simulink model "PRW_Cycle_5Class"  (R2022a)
settings: Solver=VariableStepAuto  StartTime=0.0  StopTime=simtime  RelTol=1e-3
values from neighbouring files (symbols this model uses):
  GT = SOH_p01(data_length_finish,1)    [Data_preparation.m]    (also in SimulationCycle.m = 1)
libraries: neural x183
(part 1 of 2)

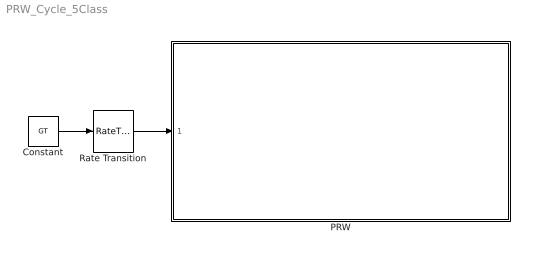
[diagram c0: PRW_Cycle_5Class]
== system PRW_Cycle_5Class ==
  Constant : Constant  Value=GT
  PRW : Subsystem
  Rate Transition : RateTransition  OutPortSampleTime=1
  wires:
  Rate Transition/1 -> PRW/1(SOH)
  Constant/1 -> Rate Transition/1

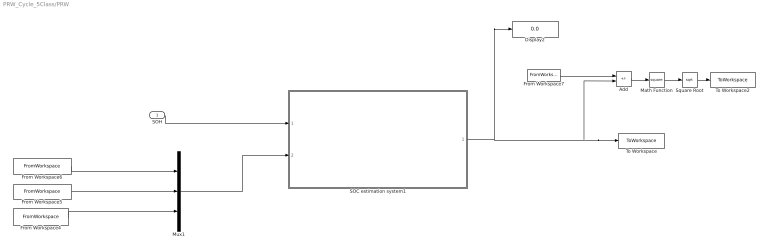
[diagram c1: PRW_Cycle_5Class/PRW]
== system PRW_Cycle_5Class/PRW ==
  SOH : Inport
  Add : Sum  Inputs=+-
  Display2 : Display
  From Workspace4 : FromWorkspace  VariableName=Temperature37
  From Workspace5 : FromWorkspace  VariableName=Voltage37  SampleTime=1
  From Workspace6 : FromWorkspace  VariableName=Current37  SampleTime=1
  From Workspace7 : FromWorkspace  VariableName=SOC_37_GT
  Math Function : Math  Operator=square
  Mux1 : Mux  Inputs=3
  SOC estimation system1 : Subsystem
  Square Root : Sqrt
  To Workspace : ToWorkspace  VariableName=SOC_37_pred  SaveFormat=Timeseries  SampleTime=-1
  To Workspace2 : ToWorkspace  VariableName=SOC_37_abserror  SampleTime=-1
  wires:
  From Workspace6/1 -> Mux1/1
  From Workspace5/1 -> Mux1/2
  From Workspace4/1 -> Mux1/3
  Mux1/1 -> SOC estimation system1/2(Input)
  SOH/1 -> SOC estimation system1/1(Input1)
  Math Function/1 -> Square Root/1
  SOC estimation system1/1(SOC) -> Display2/1, To Workspace/1, Add/2
  From Workspace7/1 -> Add/1
  Add/1 -> Math Function/1
  Square Root/1 -> To Workspace2/1

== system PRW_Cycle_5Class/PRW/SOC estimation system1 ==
  Input1 : Inport
  Input : Inport  Port=2
  Class 1 : Subsystem
  Class 2 : Subsystem
  Class 3 : Subsystem
  Class 4 : Subsystem
  Class 5 : Subsystem
  If1 : If  IfExpression=0.96<u1  ElseIfExpressions=0.92<u1&u1<=0.96  ShowElse=off
  If2 : If  IfExpression=0.9<u1&u1<=0.92  ElseIfExpressions=0.87<u1&u1<=0.9  ShowElse=off
  If3 : If  IfExpression=u1<=0.87  ShowElse=off
  Merge1 : Merge  Inputs=5
  SOC : Outport
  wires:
  If3/1 -> Class 5/Action
  If2/2 -> Class 4/Action
  Class 3/1(Output2) -> Merge1/3
  Class 2/1(Output1) -> Merge1/2
  Class 1/1(Output) -> Merge1/1
  If1/1 -> Class 1/Action
  Class 4/1(Output3) -> Merge1/4
  Input1/1 -> If3/1, If1/1, If2/1
  Class 5/1(Output4) -> Merge1/5
  Merge1/1 -> SOC/1
  If1/2 -> Class 2/Action
  If2/1 -> Class 3/Action
  Input/1 -> Class 1/1(Input), Class 2/1(Input1), Class 3/1(Input2), Class 4/1(Input3), Class 5/1(Input4)

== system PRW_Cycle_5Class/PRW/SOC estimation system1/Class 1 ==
  Input : Inport
  Action Port : ActionPort  ActionPortLabel=if(0.96<u1)
  Class 1-NARX Neural Network : Subsystem  mask{pi_input_1_delayed_1=[0.5037406483790520805854384889244101941585540771484375;0.940456819140602195972178378724493086338043212890625;-0.2518202360030123987399974794243462383747100830078125], ai_layer_2_delayed_1=0.9999911873568390063837796333245933055877685546875}
      mask prompts: pi_input_1_delayed_1 "Preprocessed initial input 1 state at timestep 0."; ai_layer_2_delayed_1 "Initial layer 2 state at timestep 0."
      mask help: NARX Neural Network
  Output : Outport
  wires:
  Class 1-NARX Neural Network/1(y) -> Output/1
  Input/1 -> Class 1-NARX Neural Network/1(x)

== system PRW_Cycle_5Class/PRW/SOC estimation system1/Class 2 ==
  Input1 : Inport
  Action Port : ActionPort  ActionPortLabel=elseif(0.92<u1&u1<=0.96)
  Class2-NARX Neural Network : Subsystem  mask{pi_input_1_delayed_1=[0.4967578681005850871343909602728672325611114501953125;0.9493670886075957771055300327134318649768829345703125;-0.57323420074349396013957402828964404761791229248046875], ai_layer_2_delayed_1=0.99999172247877510244506993331015110015869140625}
      mask prompts: pi_input_1_delayed_1 "Preprocessed initial input 1 state at timestep 0."; ai_layer_2_delayed_1 "Initial layer 2 state at timestep 0."
      mask help: NARX Neural Network
  Output1 : Outport
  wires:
  Input1/1 -> Class2-NARX Neural Network/1(x)
  Class2-NARX Neural Network/1(y) -> Output1/1

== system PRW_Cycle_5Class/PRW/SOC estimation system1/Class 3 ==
  Input2 : Inport
  Action Port : ActionPort  ActionPortLabel=if(0.9<u1&u1<=0.92)
  Class3-NARX Neural Network : Subsystem  mask{pi_input_1_delayed_1=[0.503541633873760385853302068426273763179779052734375;0.9477866061293991339908870941144414246082305908203125;-1.2699044585987255828740671859122812747955322265625], ai_layer_2_delayed_1=0.99999085582048241604979921248741447925567626953125}
      mask prompts: pi_input_1_delayed_1 "Preprocessed initial input 1 state at timestep 0."; ai_layer_2_delayed_1 "Initial layer 2 state at timestep 0."
      mask help: NARX Neural Network
  Output2 : Outport
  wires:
  Class3-NARX Neural Network/1(y) -> Output2/1
  Input2/1 -> Class3-NARX Neural Network/1(x)

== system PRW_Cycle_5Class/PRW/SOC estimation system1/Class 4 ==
  Input3 : Inport
  Action Port : ActionPort  ActionPortLabel=elseif(0.87<u1&u1<=0.9)
  Class 4-NARX Neural Network : Subsystem  mask{pi_input_1_delayed_1=[0.509984639016896945662438156432472169399261474609375;0.9369725738396628145210343063808977603912353515625;-0.6748366013071891433838800367084331810474395751953125], ai_layer_2_delayed_1=0.999984478854660352453720406629145145416259765625}
      mask prompts: pi_input_1_delayed_1 "Preprocessed initial input 1 state at timestep 0."; ai_layer_2_delayed_1 "Initial layer 2 state at timestep 0."
      mask help: NARX Neural Network
  Output3 : Outport
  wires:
  Class 4-NARX Neural Network/1(y) -> Output3/1
  Input3/1 -> Class 4-NARX Neural Network/1(x)

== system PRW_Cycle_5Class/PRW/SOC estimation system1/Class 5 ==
  Input4 : Inport
  Action Port : ActionPort  ActionPortLabel=if(u1<=0.87)
  Class5-NARX Neural Network : Subsystem  mask{pi_input_1_delayed_1=[0.5179502915004601248938342905603349208831787109375;0.9320641543877956625152592096128500998020172119140625;-0.2691648297820226076737526454962790012359619140625], ai_layer_2_delayed_1=0.999983626849760387500509750680066645145416259765625}
      mask prompts: pi_input_1_delayed_1 "Preprocessed initial input 1 state at timestep 0."; ai_layer_2_delayed_1 "Initial layer 2 state at timestep 0."
      mask help: NARX Neural Network
  Output4 : Outport
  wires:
  Class5-NARX Neural Network/1(y) -> Output4/1
  Input4/1 -> Class5-NARX Neural Network/1(x)

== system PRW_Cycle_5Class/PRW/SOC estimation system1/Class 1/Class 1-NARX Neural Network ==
  x : Inport  PortDimensions=3  SampleTime=1
  Layer 1 : Subsystem
  Layer 2 : Subsystem
  Process Input 1 : Subsystem
  Process Output 1 : Subsystem
  y : Outport  InitialOutput=0
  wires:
  x/1 -> Process Input 1/1(x)
  Process Output 1/1(y) -> y/1
  Process Input 1/1(p) -> Layer 1/1("p{1}")
  Layer 1/1("a{1}") -> [feedback1]
  [feedback1] -> Layer 2/1("a{1} ")
  Layer 2/1("a{2}") -> [feedback2], Process Output 1/1(a)
  [feedback2] -> Layer 1/2("a{2} ")

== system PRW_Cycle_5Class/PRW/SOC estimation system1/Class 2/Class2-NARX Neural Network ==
  x : Inport  PortDimensions=3  SampleTime=1
  Layer 1 : Subsystem
  Layer 2 : Subsystem
  Process Input 1 : Subsystem
  Process Output 1 : Subsystem
  y : Outport  InitialOutput=0
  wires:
  x/1 -> Process Input 1/1(x)
  Process Output 1/1(y) -> y/1
  Process Input 1/1(p) -> Layer 1/1("p{1}")
  Layer 1/1("a{1}") -> [feedback1]
  [feedback1] -> Layer 2/1("a{1} ")
  Layer 2/1("a{2}") -> [feedback2], Process Output 1/1(a)
  [feedback2] -> Layer 1/2("a{2} ")

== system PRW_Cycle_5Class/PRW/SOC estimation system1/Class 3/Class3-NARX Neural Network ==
  x : Inport  PortDimensions=3  SampleTime=1
  Layer 1 : Subsystem
  Layer 2 : Subsystem
  Process Input 1 : Subsystem
  Process Output 1 : Subsystem
  y : Outport  InitialOutput=0
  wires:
  x/1 -> Process Input 1/1(x)
  Process Output 1/1(y) -> y/1
  Process Input 1/1(p) -> Layer 1/1("p{1}")
  Layer 1/1("a{1}") -> [feedback1]
  [feedback1] -> Layer 2/1("a{1} ")
  Layer 2/1("a{2}") -> [feedback2], Process Output 1/1(a)
  [feedback2] -> Layer 1/2("a{2} ")

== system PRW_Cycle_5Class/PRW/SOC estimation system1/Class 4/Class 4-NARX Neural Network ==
  x : Inport  PortDimensions=3  SampleTime=1
  Layer 1 : Subsystem
  Layer 2 : Subsystem
  Process Input 1 : Subsystem
  Process Output 1 : Subsystem
  y : Outport  InitialOutput=0
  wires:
  x/1 -> Process Input 1/1(x)
  Process Output 1/1(y) -> y/1
  Process Input 1/1(p) -> Layer 1/1("p{1}")
  Layer 1/1("a{1}") -> [feedback1]
  [feedback1] -> Layer 2/1("a{1} ")
  Layer 2/1("a{2}") -> [feedback2], Process Output 1/1(a)
  [feedback2] -> Layer 1/2("a{2} ")

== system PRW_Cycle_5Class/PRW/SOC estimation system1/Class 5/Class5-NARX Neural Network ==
  x : Inport  PortDimensions=3  SampleTime=1
  Layer 1 : Subsystem
  Layer 2 : Subsystem
  Process Input 1 : Subsystem
  Process Output 1 : Subsystem
  y : Outport  InitialOutput=0
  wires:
  x/1 -> Process Input 1/1(x)
  Process Output 1/1(y) -> y/1
  Process Input 1/1(p) -> Layer 1/1("p{1}")
  Layer 1/1("a{1}") -> [feedback1]
  [feedback1] -> Layer 2/1("a{1} ")
  Layer 2/1("a{2}") -> [feedback2], Process Output 1/1(a)
  [feedback2] -> Layer 1/2("a{2} ")

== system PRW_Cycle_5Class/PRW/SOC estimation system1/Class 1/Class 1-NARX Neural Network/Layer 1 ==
  "p{1}" : Inport  PortDimensions=3  SampleTime=1
  "a{2} " : Inport  Port=2  PortDimensions=1  SampleTime=1
  Delays 1 : Subsystem
  Delays 2 : Subsystem
  "IW{1,1}" : Subsystem
  "LW{1,2}" : Subsystem
  "b{1}" : Constant  Value=[2.34272603015963820638489778502844274044036865234375;-1.83098571478465554918102498049847781658172607421875;-0.79131154125893576889438918442465364933013916015625;-1.2076273263687624659468156096409074962139129638671875;0.84071386902655909079129514793748967349529266357421875;-0.53056878404548457606182410017936490476131439208984375;-0.0240383625943490740473063027593525475822389125823974609375;0.16604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
  netsum : Sum  Inputs=3  InputSameDT=on  SaturateOnIntegerOverflow=on
  tansig : neural/Transfer Functions/tansig
  "a{1}" : Outport  InitialOutput=[0;0;0;0;0;0;0;0;0;0;0;0;0;0;0]
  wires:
  "p{1}"/1 -> Delays 1/1("p{1}")
  Delays 1/1("pd{1,1}") -> "IW{1,1}"/1("pd{1,1}")
  "IW{1,1}"/1("iz{1,1}") -> netsum/1
  "a{2} "/1 -> Delays 2/1("p{1}")
  Delays 2/1("pd{1,2}") -> "LW{1,2}"/1("ad{1,2}")
  "LW{1,2}"/1("lz{1,2}") -> netsum/2
  "b{1}"/1 -> netsum/3
  netsum/1 -> tansig/1
  tansig/1 -> "a{1}"/1

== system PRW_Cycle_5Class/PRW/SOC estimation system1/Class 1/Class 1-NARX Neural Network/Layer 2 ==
  "a{1} " : Inport  PortDimensions=15  SampleTime=1
  Delays 1 : Subsystem
  "LW{2,1}" : Subsystem
  "b{2}" : Constant  Value=-0.2610570456976468722842810166184790432453155517578125
  netsum : Sum  Inputs=2  InputSameDT=on  SaturateOnIntegerOverflow=on
  purelin : neural/Transfer Functions/purelin
  "a{2}" : Outport  InitialOutput=0
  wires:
  "a{1} "/1 -> Delays 1/1("p{2}")
  Delays 1/1("pd{2,1}") -> "LW{2,1}"/1("ad{2,1}")
  "LW{2,1}"/1("lz{2,1}") -> netsum/1
  "b{2}"/1 -> netsum/2
  netsum/1 -> purelin/1
  purelin/1 -> "a{2}"/1

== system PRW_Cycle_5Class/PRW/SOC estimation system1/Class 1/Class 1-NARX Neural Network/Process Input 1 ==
  x : Inport  PortDimensions=3  SampleTime=1
  mapminmax : neural/Processing Functions/mapminmax  xmin=[-4.82500000000000017763568394003;2.50570000000000003836930773105;17.1380000000000016768808563938]  xmax=[1.5909999999999999698019337302;4.16500000000000003552713678801;25.1039999999999992041921359487]  ymin=-1  ymax=1
  p : Outport  PortDimensions=3  SampleTime=1
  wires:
  x/1 -> mapminmax/1
  mapminmax/1 -> p/1

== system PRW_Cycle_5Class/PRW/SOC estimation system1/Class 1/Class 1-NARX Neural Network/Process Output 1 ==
  a : Inport  PortDimensions=1  SampleTime=1
  mapminmax_reverse : neural/Processing Functions/mapminmax_reverse  xmin=-2.62341179120179950748424461959e-06  xmax=1.00000440635255594123975697585  ymin=-1  ymax=1
  y : Outport  PortDimensions=1  SampleTime=1
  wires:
  a/1 -> mapminmax_reverse/1
  mapminmax_reverse/1 -> y/1

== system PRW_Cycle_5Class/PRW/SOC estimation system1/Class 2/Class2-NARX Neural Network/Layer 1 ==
  "p{1}" : Inport  PortDimensions=3  SampleTime=1
  "a{2} " : Inport  Port=2  PortDimensions=1  SampleTime=1
  Delays 1 : Subsystem
  Delays 2 : Subsystem
  "IW{1,1}" : Subsystem
  "LW{1,2}" : Subsystem
  "b{1}" : Constant  Value=[2.123679128509173619221428452874533832073211669921875;-2.87621199885181422217783619998954236507415771484375;-0.54420836494168567387674784185946919023990631103515625;-0.5394065908795988573132262899889610707759857177734375;0.85139936745729760669831875929958187043666839599609375;-1.1563643607811477931335275570745579898357391357421875;-0.61089692546734919442741329476120881736278533935546875;-0.197690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
  netsum : Sum  Inputs=3  InputSameDT=on  SaturateOnIntegerOverflow=on
  tansig : neural/Transfer Functions/tansig
  "a{1}" : Outport  InitialOutput=[0;0;0;0;0;0;0;0;0;0;0;0;0;0;0;0]
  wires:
  "p{1}"/1 -> Delays 1/1("p{1}")
  Delays 1/1("pd{1,1}") -> "IW{1,1}"/1("pd{1,1}")
  "IW{1,1}"/1("iz{1,1}") -> netsum/1
  "a{2} "/1 -> Delays 2/1("p{1}")
  Delays 2/1("pd{1,2}") -> "LW{1,2}"/1("ad{1,2}")
  "LW{1,2}"/1("lz{1,2}") -> netsum/2
  "b{1}"/1 -> netsum/3
  netsum/1 -> tansig/1
  tansig/1 -> "a{1}"/1

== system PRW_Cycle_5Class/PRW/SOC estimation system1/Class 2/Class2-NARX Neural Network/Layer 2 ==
  "a{1} " : Inport  PortDimensions=16  SampleTime=1
  Delays 1 : Subsystem
  "LW{2,1}" : Subsystem
  "b{2}" : Constant  Value=0.1380564376019000061290853409445844590663909912109375
  netsum : Sum  Inputs=2  InputSameDT=on  SaturateOnIntegerOverflow=on
  purelin : neural/Transfer Functions/purelin
  "a{2}" : Outport  InitialOutput=0
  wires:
  "a{1} "/1 -> Delays 1/1("p{2}")
  Delays 1/1("pd{2,1}") -> "LW{2,1}"/1("ad{2,1}")
  "LW{2,1}"/1("lz{2,1}") -> netsum/1
  "b{2}"/1 -> netsum/2
  netsum/1 -> purelin/1
  purelin/1 -> "a{2}"/1

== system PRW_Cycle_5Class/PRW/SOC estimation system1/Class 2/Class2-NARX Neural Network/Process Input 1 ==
  x : Inport  PortDimensions=3  SampleTime=1
  mapminmax : neural/Processing Functions/mapminmax  xmin=[-4.73300000000000054001247917768;2.63719999999999998863131622784;17.8219999999999991757704265183]  xmax=[1.59000000000000007993605777301;4.15399999999999991473487170879;28.5820000000000007389644451905]  ymin=-1  ymax=1
  p : Outport  PortDimensions=3  SampleTime=1
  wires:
  x/1 -> mapminmax/1
  mapminmax/1 -> p/1

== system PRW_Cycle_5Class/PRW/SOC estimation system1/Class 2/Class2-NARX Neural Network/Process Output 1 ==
  a : Inport  PortDimensions=1  SampleTime=1
  mapminmax_reverse : neural/Processing Functions/mapminmax_reverse  xmin=-3.32617917940104848405083806662e-06  xmax=1.00000413879150817919594373961  ymin=-1  ymax=1
  y : Outport  PortDimensions=1  SampleTime=1
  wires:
  a/1 -> mapminmax_reverse/1
  mapminmax_reverse/1 -> y/1

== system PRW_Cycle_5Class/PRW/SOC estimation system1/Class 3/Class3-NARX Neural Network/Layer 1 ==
  "p{1}" : Inport  PortDimensions=3  SampleTime=1
  "a{2} " : Inport  Port=2  PortDimensions=1  SampleTime=1
  Delays 1 : Subsystem
  Delays 2 : Subsystem
  "IW{1,1}" : Subsystem
  "LW{1,2}" : Subsystem
  "b{1}" : Constant  Value=[-1.93346371221756019309623297885991632938385009765625;1.7923652112547914239115698364912532269954681396484375;1.1238522489621971534035083095659501850605010986328125;0.323356733008480279334406759517150931060314178466796875;0.76493308526969572280762577065615914762020111083984375;-0.351089604850296443938617585445172153413295745849609375;0.33583797370279000471526842375169508159160614013671875;-0.46332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
  netsum : Sum  Inputs=3  InputSameDT=on  SaturateOnIntegerOverflow=on
  tansig : neural/Transfer Functions/tansig
  "a{1}" : Outport  InitialOutput=[0;0;0;0;0;0;0;0;0;0;0;0;0;0;0]
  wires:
  "p{1}"/1 -> Delays 1/1("p{1}")
  Delays 1/1("pd{1,1}") -> "IW{1,1}"/1("pd{1,1}")
  "IW{1,1}"/1("iz{1,1}") -> netsum/1
  "a{2} "/1 -> Delays 2/1("p{1}")
  Delays 2/1("pd{1,2}") -> "LW{1,2}"/1("ad{1,2}")
  "LW{1,2}"/1("lz{1,2}") -> netsum/2
  "b{1}"/1 -> netsum/3
  netsum/1 -> tansig/1
  tansig/1 -> "a{1}"/1

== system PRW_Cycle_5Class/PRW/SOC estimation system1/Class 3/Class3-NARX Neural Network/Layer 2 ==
  "a{1} " : Inport  PortDimensions=15  SampleTime=1
  Delays 1 : Subsystem
  "LW{2,1}" : Subsystem
  "b{2}" : Constant  Value=0.272834520121191526076387390276067890226840972900390625
  netsum : Sum  Inputs=2  InputSameDT=on  SaturateOnIntegerOverflow=on
  purelin : neural/Transfer Functions/purelin
  "a{2}" : Outport  InitialOutput=0
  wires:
  "a{1} "/1 -> Delays 1/1("p{2}")
  Delays 1/1("pd{2,1}") -> "LW{2,1}"/1("ad{2,1}")
  "LW{2,1}"/1("lz{2,1}") -> netsum/1
  "b{2}"/1 -> netsum/2
  netsum/1 -> purelin/1
  purelin/1 -> "a{2}"/1

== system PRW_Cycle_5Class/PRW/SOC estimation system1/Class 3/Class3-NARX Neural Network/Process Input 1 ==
  x : Inport  PortDimensions=3  SampleTime=1
  mapminmax : neural/Processing Functions/mapminmax  xmin=[-4.77700000000000013500311979442;2.6570000000000000284217094304;21.4740000000000001989519660128]  xmax=[1.57600000000000006750155989721;4.15470000000000005968558980385;31.5220000000000020179413695587]  ymin=-1  ymax=1
  p : Outport  PortDimensions=3  SampleTime=1
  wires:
  x/1 -> mapminmax/1
  mapminmax/1 -> p/1

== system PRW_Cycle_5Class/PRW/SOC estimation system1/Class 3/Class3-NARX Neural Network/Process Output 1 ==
  a : Inport  PortDimensions=1  SampleTime=1
  mapminmax_reverse : neural/Processing Functions/mapminmax_reverse  xmin=-3.07535918984610110574521267546e-06  xmax=1.00000457212472371182343522378  ymin=-1  ymax=1
  y : Outport  PortDimensions=1  SampleTime=1
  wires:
  a/1 -> mapminmax_reverse/1
  mapminmax_reverse/1 -> y/1

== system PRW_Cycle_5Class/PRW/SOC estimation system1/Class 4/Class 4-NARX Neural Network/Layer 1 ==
  "p{1}" : Inport  PortDimensions=3  SampleTime=1
  "a{2} " : Inport  Port=2  PortDimensions=1  SampleTime=1
  Delays 1 : Subsystem
  Delays 2 : Subsystem
  "IW{1,1}" : Subsystem
  "LW{1,2}" : Subsystem
  "b{1}" : Constant  Value=[-2.688444044962437828871770761907100677490234375;0.858381113224772729353162503684870898723602294921875;-2.222715747204785596835563410422764718532562255859375;1.3209762857863693863436083120177499949932098388671875;-0.8915787953875426996575015436974354088306427001953125;-0.88615966223780884281069347707671113312244415283203125;0.280218393721010927688297442728071473538875579833984375;0.21524348971530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
  netsum : Sum  Inputs=3  InputSameDT=on  SaturateOnIntegerOverflow=on
  tansig : neural/Transfer Functions/tansig
  "a{1}" : Outport  InitialOutput=[0;0;0;0;0;0;0;0;0;0;0;0;0;0;0]
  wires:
  "p{1}"/1 -> Delays 1/1("p{1}")
  Delays 1/1("pd{1,1}") -> "IW{1,1}"/1("pd{1,1}")
  "IW{1,1}"/1("iz{1,1}") -> netsum/1
  "a{2} "/1 -> Delays 2/1("p{1}")
  Delays 2/1("pd{1,2}") -> "LW{1,2}"/1("ad{1,2}")
  "LW{1,2}"/1("lz{1,2}") -> netsum/2
  "b{1}"/1 -> netsum/3
  netsum/1 -> tansig/1
  tansig/1 -> "a{1}"/1

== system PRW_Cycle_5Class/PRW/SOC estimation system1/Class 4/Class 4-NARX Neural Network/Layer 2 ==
  "a{1} " : Inport  PortDimensions=15  SampleTime=1
  Delays 1 : Subsystem
  "LW{2,1}" : Subsystem
  "b{2}" : Constant  Value=0.045626078950611735629561138694043620489537715911865234375
  netsum : Sum  Inputs=2  InputSameDT=on  SaturateOnIntegerOverflow=on
  purelin : neural/Transfer Functions/purelin
  "a{2}" : Outport  InitialOutput=0
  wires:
  "a{1} "/1 -> Delays 1/1("p{2}")
  Delays 1/1("pd{2,1}") -> "LW{2,1}"/1("ad{2,1}")
  "LW{2,1}"/1("lz{2,1}") -> netsum/1
  "b{2}"/1 -> netsum/2
  netsum/1 -> purelin/1
  purelin/1 -> "a{2}"/1

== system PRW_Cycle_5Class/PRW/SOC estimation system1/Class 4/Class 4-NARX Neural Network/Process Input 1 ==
  x : Inport  PortDimensions=3  SampleTime=1
  mapminmax : neural/Processing Functions/mapminmax  xmin=[-4.91600000000000036948222259525;2.64660000000000028563817977556;18.5259999999999998010480339872]  xmax=[1.59400000000000008348877145181;4.16340000000000021174173525651;28.3180000000000013926637620898]  ymin=-1  ymax=1
  p : Outport  PortDimensions=3  SampleTime=1
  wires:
  x/1 -> mapminmax/1
  mapminmax/1 -> p/1

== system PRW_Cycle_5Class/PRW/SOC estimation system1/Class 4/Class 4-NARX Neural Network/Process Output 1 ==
  a : Inport  PortDimensions=1  SampleTime=1
  mapminmax_reverse : neural/Processing Functions/mapminmax_reverse  xmin=-4.21949321457851519659313158095e-06  xmax=1.00000776066564278643511443079  ymin=-1  ymax=1
  y : Outport  PortDimensions=1  SampleTime=1
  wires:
  a/1 -> mapminmax_reverse/1
  mapminmax_reverse/1 -> y/1

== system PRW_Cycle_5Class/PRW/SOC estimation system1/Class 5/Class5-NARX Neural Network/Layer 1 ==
  "p{1}" : Inport  PortDimensions=3  SampleTime=1
  "a{2} " : Inport  Port=2  PortDimensions=1  SampleTime=1
  Delays 1 : Subsystem
  Delays 2 : Subsystem
  "IW{1,1}" : Subsystem
  "LW{1,2}" : Subsystem
  "b{1}" : Constant  Value=[-1.9239326886795684590225619103875942528247833251953125;-1.4156259333430829538968964698142372071743011474609375;-1.8809744346361843003734293233719654381275177001953125;-1.106968201899322767900457620271481573581695556640625;1.16695809702027997190043606678955256938934326171875;1.0579085603689832861817876619170419871807098388671875;0.33221840417104486764543480603606440126895904541015625;-0.035398306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
  netsum : Sum  Inputs=3  InputSameDT=on  SaturateOnIntegerOverflow=on
  tansig : neural/Transfer Functions/tansig
  "a{1}" : Outport  InitialOutput=[0;0;0;0;0;0;0;0;0;0;0;0;0;0;0;0;0;0]
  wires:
  "p{1}"/1 -> Delays 1/1("p{1}")
  Delays 1/1("pd{1,1}") -> "IW{1,1}"/1("pd{1,1}")
  "IW{1,1}"/1("iz{1,1}") -> netsum/1
  "a{2} "/1 -> Delays 2/1("p{1}")
  Delays 2/1("pd{1,2}") -> "LW{1,2}"/1("ad{1,2}")
  "LW{1,2}"/1("lz{1,2}") -> netsum/2
  "b{1}"/1 -> netsum/3
  netsum/1 -> tansig/1
  tansig/1 -> "a{1}"/1

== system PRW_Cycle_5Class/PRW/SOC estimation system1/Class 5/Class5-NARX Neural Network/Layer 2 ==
  "a{1} " : Inport  PortDimensions=18  SampleTime=1
  Delays 1 : Subsystem
  "LW{2,1}" : Subsystem
  "b{2}" : Constant  Value=0.2439901834476533026840883167096762917935848236083984375
  netsum : Sum  Inputs=2  InputSameDT=on  SaturateOnIntegerOverflow=on
  purelin : neural/Transfer Functions/purelin
  "a{2}" : Outport  InitialOutput=0
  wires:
  "a{1} "/1 -> Delays 1/1("p{2}")
  Delays 1/1("pd{2,1}") -> "LW{2,1}"/1("ad{2,1}")
  "LW{2,1}"/1("lz{2,1}") -> netsum/1
  "b{2}"/1 -> netsum/2
  netsum/1 -> purelin/1
  purelin/1 -> "a{2}"/1

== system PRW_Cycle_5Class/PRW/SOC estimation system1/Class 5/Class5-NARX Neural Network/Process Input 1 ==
  x : Inport  PortDimensions=3  SampleTime=1
  mapminmax : neural/Processing Functions/mapminmax  xmin=[-4.94800000000000039790393202566;2.6339000000000001300293206441;17.1340000000000003410605131648]  xmax=[1.57000000000000006217248937901;4.16769999999999996020960679743;25.3000000000000007105427357601]  ymin=-1  ymax=1
  p : Outport  PortDimensions=3  SampleTime=1
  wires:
  x/1 -> mapminmax/1
  mapminmax/1 -> p/1

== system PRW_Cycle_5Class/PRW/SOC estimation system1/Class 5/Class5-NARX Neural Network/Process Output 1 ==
  a : Inport  PortDimensions=1  SampleTime=1
  mapminmax_reverse : neural/Processing Functions/mapminmax_reverse  xmin=-3.87764264893447179729721319141e-06  xmax=1.0000081866738852465203990505  ymin=-1  ymax=1
  y : Outport  PortDimensions=1  SampleTime=1
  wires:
  a/1 -> mapminmax_reverse/1
  mapminmax_reverse/1 -> y/1

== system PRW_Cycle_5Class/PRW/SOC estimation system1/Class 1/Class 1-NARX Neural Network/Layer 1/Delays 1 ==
  "p{1}" : Inport  PortDimensions=3  SampleTime=1
  Delay 1 : UnitDelay  InitialCondition=pi_input_1_delayed_1
  mux : Mux  Inputs=2
  "pd{1,1}" : Outport
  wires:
  "p{1}"/1 -> Delay 1/1, mux/1
  Delay 1/1 -> mux/2
  mux/1 -> "pd{1,1}"/1

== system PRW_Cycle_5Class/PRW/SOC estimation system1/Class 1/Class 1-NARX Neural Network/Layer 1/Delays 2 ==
  "p{1}" : Inport  PortDimensions=1  SampleTime=1
  Delay 1 : UnitDelay  InitialCondition=ai_layer_2_delayed_1
  mux : Mux  Inputs=1
  "pd{1,2}" : Outport
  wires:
  "p{1}"/1 -> Delay 1/1
  Delay 1/1 -> mux/1
  mux/1 -> "pd{1,2}"/1

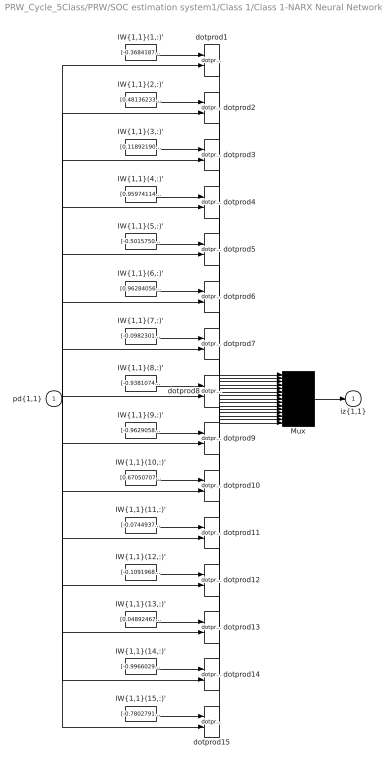
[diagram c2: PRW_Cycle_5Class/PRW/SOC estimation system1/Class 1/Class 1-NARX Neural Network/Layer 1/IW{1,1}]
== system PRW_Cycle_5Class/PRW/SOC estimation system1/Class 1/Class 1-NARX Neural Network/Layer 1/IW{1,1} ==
  "pd{1,1}" : Inport  PortDimensions=6  SampleTime=1
  "IW{1,1}(1,:)'" : Constant  Value=[-0.36841871672555603911547450479702092707157135009765625;0.95481863811988365586813642948982305824756622314453125;0.226878529936702599822950787711306475102901458740234375;0.036258766201381888161225930389264249242842197418212890625;0.3238678699587700382522825748310424387454986572265625;-0.84200791510325945221637766735511831939220428466796875]
  "IW{1,1}(10,:)'" : Constant  Value=[0.67050707720070523709665621936437673866748809814453125;0.882956797146274841026070134830661118030548095703125;-0.90123173513004661838721176536637358367443084716796875;0.89515060785826994216307639362639747560024261474609375;-0.805115591223422466526926655205897986888885498046875;-0.2593277792147092863928037331788800656795501708984375]
  "IW{1,1}(11,:)'" : Constant  Value=[-0.0744937388110009646169373809243552386760711669921875;0.91481150331324145863476360318600200116634368896484375;-0.0033589550935993598736184484465638888650573790073394775390625;0.09387686590177278522784121150834835134446620941162109375;-0.99451251190708223059999681936460547149181365966796875;-0.0003307952570151217433665202793946491510723717510700225830078125]
  "IW{1,1}(12,:)'" : Constant  Value=[-0.10919681936643919895058019164935103617608547210693359375;0.50465640273350442779332070131204091012477874755859375;0.00167935474555881941553792113808185604284517467021942138671875;0.090898075716160431358758842179668135941028594970703125;-0.421892519785072861449037873171619139611721038818359375;0.004083310809217589355812894069686080911196768283843994140625]
  "IW{1,1}(13,:)'" : Constant  Value=[0.048924672243263016280234722898967447690665721893310546875;-0.53987449057316327927225074745365418493747711181640625;0.00170226104659932341023331758833592175506055355072021484375;-0.058328940083118230308656393390265293419361114501953125;0.57776802472895305573530322362785227596759796142578125;-0.00015032127929270978146554516019506309021380729973316192626953125]
  "IW{1,1}(14,:)'" : Constant  Value=[-0.99660291683138291229937522075488232076168060302734375;0.5911312952433938061602702873642556369304656982421875;1.14540739846979366944879075163044035434722900390625;-0.3381076514679877131897001163451932370662689208984375;0.45894832786268346946911833583726547658443450927734375;-0.70176558995015925201954587464570067822933197021484375]
  "IW{1,1}(15,:)'" : Constant  Value=[-0.7802791008156886309876654195250011980533599853515625;1.0534129951958177695559015774051658809185028076171875;-0.03448938205268679835224787666447809897363185882568359375;0.94691798651251091190061970337410457432270050048828125;0.0231481724065754346231216231899452395737171173095703125;-0.5027468755563602176295034951181150972843170166015625]
  "IW{1,1}(2,:)'" : Constant  Value=[0.481362338278815193870485700244898907840251922607421875;-1.50652710762162467261759957182221114635467529296875;-0.2359262305730511488643941220288979820907115936279296875;-0.1406423235510661229330509058854659087955951690673828125;0.1819515858690983478584968224822659976780414581298828125;0.86381133633920403891437445054179988801479339599609375]
  "IW{1,1}(3,:)'" : Constant  Value=[0.11892190500532838492997456114608212374150753021240234375;-0.24493184734591633144873412675224244594573974609375;-0.00451567345059881997126893793392810039222240447998046875;-0.08059998953516155084653149742734967730939388275146484375;0.07911717353434512267629230564125464297831058502197265625;-0.00710306128001607188504618051183570059947669506072998046875]
  "IW{1,1}(4,:)'" : Constant  Value=[0.95974114664550247422170059508061967790126800537109375;-0.8796676994389194259582609447534196078777313232421875;0.9728248784750912481200657566660083830356597900390625;-0.70361057504988477884211306445649825036525726318359375;0.6194834636783788095470981716061942279338836669921875;0.61913161067906596901622151563060469925403594970703125]
  "IW{1,1}(5,:)'" : Constant  Value=[-0.50157500574550883953861557529307901859283447265625;-0.375530160518852185180804781339247711002826690673828125;0.01501545548960662480875161151061547570861876010894775390625;0.757425535532789684367571680922992527484893798828125;-0.77182219089220105434634433549945242702960968017578125;-0.0759994756633779744436907321869512088596820831298828125]
  "IW{1,1}(6,:)'" : Constant  Value=[0.9628405697273880736730689022806473076343536376953125;-0.632510343955252185565996114746667444705963134765625;0.35396101720878470064945986450766213238239288330078125;-0.60680374926630076259925772319547832012176513671875;0.177448918867727456483152082000742666423320770263671875;0.9817426047833206492754243299714289605617523193359375]
  "IW{1,1}(7,:)'" : Constant  Value=[-0.09823010496840246796868001410985016264021396636962890625;-1.185310142409820688413901734747923910617828369140625;0.1908758613743539445106733865031856112182140350341796875;-1.1914761953630537139048328754142858088016510009765625;0.39827398536536140483121926081366837024688720703125;0.90973345961705021078813615531544201076030731201171875]
  "IW{1,1}(8,:)'" : Constant  Value=[-0.93810741037665390518185404289397411048412322998046875;-1.2595077433783707920866845597629435360431671142578125;-0.78652190025548751606265795999206602573394775390625;-0.7895482370616810907648641659761779010295867919921875;0.24445192827118944478570483624935150146484375;0.34046059489771918205036627114168368279933929443359375]
  "IW{1,1}(9,:)'" : Constant  Value=[-0.962905875728648386058239339035935699939727783203125;-0.99822741054854535747153931879438459873199462890625;1.4514584750111370059499904527910985052585601806640625;-0.338753693920172793685452461431850679218769073486328125;-0.2495656714555981314784816049723303876817226409912109375;-0.0823827548058631842220478347371681593358516693115234375]
  Mux : Mux  Inputs=15
  dotprod{1..15} (15 alike) : neural/Weight Functions/dotprod
  "iz{1,1}" : Outport
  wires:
  "IW{1,1}(1,:)'"/1 -> dotprod1/1
  "pd{1,1}"/1 -> dotprod1/2, dotprod2/2, dotprod3/2, dotprod4/2, dotprod5/2, dotprod6/2, dotprod7/2, dotprod8/2, dotprod9/2, dotprod10/2, dotprod11/2, dotprod12/2, dotprod13/2, dotprod14/2, dotprod15/2
  dotprod1/1 -> Mux/1
  "IW{1,1}(2,:)'"/1 -> dotprod2/1
  dotprod2/1 -> Mux/2
  "IW{1,1}(3,:)'"/1 -> dotprod3/1
  dotprod3/1 -> Mux/3
  "IW{1,1}(4,:)'"/1 -> dotprod4/1
  dotprod4/1 -> Mux/4
  "IW{1,1}(5,:)'"/1 -> dotprod5/1
  dotprod5/1 -> Mux/5
  "IW{1,1}(6,:)'"/1 -> dotprod6/1
  dotprod6/1 -> Mux/6
  "IW{1,1}(7,:)'"/1 -> dotprod7/1
  dotprod7/1 -> Mux/7
  "IW{1,1}(8,:)'"/1 -> dotprod8/1
  dotprod8/1 -> Mux/8
  "IW{1,1}(9,:)'"/1 -> dotprod9/1
  dotprod9/1 -> Mux/9
  "IW{1,1}(10,:)'"/1 -> dotprod10/1
  dotprod10/1 -> Mux/10
  "IW{1,1}(11,:)'"/1 -> dotprod11/1
  dotprod11/1 -> Mux/11
  "IW{1,1}(12,:)'"/1 -> dotprod12/1
  dotprod12/1 -> Mux/12
  "IW{1,1}(13,:)'"/1 -> dotprod13/1
  dotprod13/1 -> Mux/13
  "IW{1,1}(14,:)'"/1 -> dotprod14/1
  dotprod14/1 -> Mux/14
  "IW{1,1}(15,:)'"/1 -> dotprod15/1
  dotprod15/1 -> Mux/15
  Mux/1 -> "iz{1,1}"/1

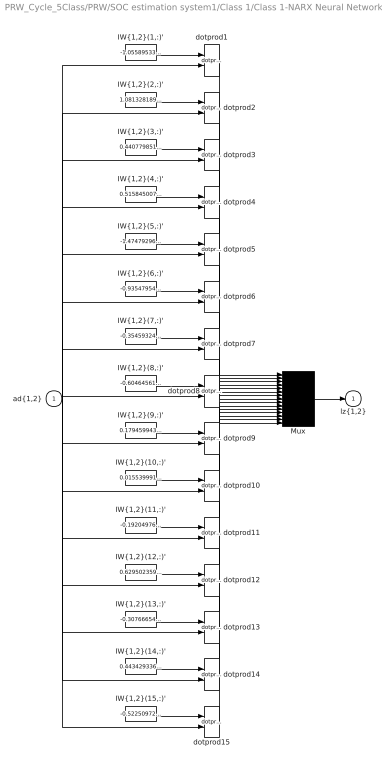
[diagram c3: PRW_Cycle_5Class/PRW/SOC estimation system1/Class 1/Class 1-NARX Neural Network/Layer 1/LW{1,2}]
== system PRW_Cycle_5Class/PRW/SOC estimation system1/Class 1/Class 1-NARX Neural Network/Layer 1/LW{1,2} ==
  "ad{1,2}" : Inport  PortDimensions=1  SampleTime=1
  "IW{1,2}(1,:)'" : Constant  Value=-1.0558953399790829141835502014146186411380767822265625
  "IW{1,2}(10,:)'" : Constant  Value=0.0155399911340668960002542320353313698433339595794677734375
  "IW{1,2}(11,:)'" : Constant  Value=-0.1920497660372149917318296274970634840428829193115234375
  "IW{1,2}(12,:)'" : Constant  Value=0.62950235962305978176800635992549359798431396484375
  "IW{1,2}(13,:)'" : Constant  Value=-0.30766654353943623245726257664500735700130462646484375
  "IW{1,2}(14,:)'" : Constant  Value=0.443429336021788522703701573846046812832355499267578125
  "IW{1,2}(15,:)'" : Constant  Value=-0.52250972552172625373856362784863449633121490478515625
  "IW{1,2}(2,:)'" : Constant  Value=1.08132818981622680354348631226457655429840087890625
  "IW{1,2}(3,:)'" : Constant  Value=0.440779851117324483755766095782746560871601104736328125
  "IW{1,2}(4,:)'" : Constant  Value=0.51584500712902159325068396356073208153247833251953125
  "IW{1,2}(5,:)'" : Constant  Value=-1.47479296662152048469351939274929463863372802734375
  "IW{1,2}(6,:)'" : Constant  Value=-0.935479542831488597443012622534297406673431396484375
  "IW{1,2}(7,:)'" : Constant  Value=-0.354593245240020948916281895435531623661518096923828125
  "IW{1,2}(8,:)'" : Constant  Value=-0.6046456148812133779557598245446570217609405517578125
  "IW{1,2}(9,:)'" : Constant  Value=0.1794599438126181223385202656572801060974597930908203125
  Mux : Mux  Inputs=15
  dotprod{1..15} (15 alike) : neural/Weight Functions/dotprod
  "lz{1,2}" : Outport
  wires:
  "IW{1,2}(1,:)'"/1 -> dotprod1/1
  "ad{1,2}"/1 -> dotprod1/2, dotprod2/2, dotprod3/2, dotprod4/2, dotprod5/2, dotprod6/2, dotprod7/2, dotprod8/2, dotprod9/2, dotprod10/2, dotprod11/2, dotprod12/2, dotprod13/2, dotprod14/2, dotprod15/2
  dotprod1/1 -> Mux/1
  "IW{1,2}(2,:)'"/1 -> dotprod2/1
  dotprod2/1 -> Mux/2
  "IW{1,2}(3,:)'"/1 -> dotprod3/1
  dotprod3/1 -> Mux/3
  "IW{1,2}(4,:)'"/1 -> dotprod4/1
  dotprod4/1 -> Mux/4
  "IW{1,2}(5,:)'"/1 -> dotprod5/1
  dotprod5/1 -> Mux/5
  "IW{1,2}(6,:)'"/1 -> dotprod6/1
  dotprod6/1 -> Mux/6
  "IW{1,2}(7,:)'"/1 -> dotprod7/1
  dotprod7/1 -> Mux/7
  "IW{1,2}(8,:)'"/1 -> dotprod8/1
  dotprod8/1 -> Mux/8
  "IW{1,2}(9,:)'"/1 -> dotprod9/1
  dotprod9/1 -> Mux/9
  "IW{1,2}(10,:)'"/1 -> dotprod10/1
  dotprod10/1 -> Mux/10
  "IW{1,2}(11,:)'"/1 -> dotprod11/1
  dotprod11/1 -> Mux/11
  "IW{1,2}(12,:)'"/1 -> dotprod12/1
  dotprod12/1 -> Mux/12
  "IW{1,2}(13,:)'"/1 -> dotprod13/1
  dotprod13/1 -> Mux/13
  "IW{1,2}(14,:)'"/1 -> dotprod14/1
  dotprod14/1 -> Mux/14
  "IW{1,2}(15,:)'"/1 -> dotprod15/1
  dotprod15/1 -> Mux/15
  Mux/1 -> "lz{1,2}"/1

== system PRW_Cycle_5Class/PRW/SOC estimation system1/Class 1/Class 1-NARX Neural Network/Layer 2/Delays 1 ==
  "p{2}" : Inport  PortDimensions=15  SampleTime=1
  mux : Mux  Inputs=1
  "pd{2,1}" : Outport
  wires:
  "p{2}"/1 -> mux/1
  mux/1 -> "pd{2,1}"/1

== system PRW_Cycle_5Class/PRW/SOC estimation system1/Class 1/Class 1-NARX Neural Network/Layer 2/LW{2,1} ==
  "ad{2,1}" : Inport  PortDimensions=15  SampleTime=1
  "IW{2,1}(1,:)'" : Constant  Value=[-0.4054339128384827350970454062917269766330718994140625;-0.150291660026959761342624233293463476002216339111328125;0.399718217310838286326912793811061419546604156494140625;3.55968054837466467703495365260124572159838862717151641845703125e-05;-0.0023970249922561893095307450352038358687423169612884521484375;-0.000111633850285505030063178122379241585804265923798084259033203125;-8.764101469894136078268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
  Mux : Mux  Inputs=1
  dotprod1 : neural/Weight Functions/dotprod
  "lz{2,1}" : Outport
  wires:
  "IW{2,1}(1,:)'"/1 -> dotprod1/1
  "ad{2,1}"/1 -> dotprod1/2
  dotprod1/1 -> Mux/1
  Mux/1 -> "lz{2,1}"/1

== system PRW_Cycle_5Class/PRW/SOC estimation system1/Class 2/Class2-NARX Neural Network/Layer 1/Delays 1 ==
  "p{1}" : Inport  PortDimensions=3  SampleTime=1
  Delay 1 : UnitDelay  InitialCondition=pi_input_1_delayed_1
  mux : Mux  Inputs=2
  "pd{1,1}" : Outport
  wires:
  "p{1}"/1 -> Delay 1/1, mux/1
  Delay 1/1 -> mux/2
  mux/1 -> "pd{1,1}"/1

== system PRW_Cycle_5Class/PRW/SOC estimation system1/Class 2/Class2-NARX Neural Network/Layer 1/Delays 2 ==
  "p{1}" : Inport  PortDimensions=1  SampleTime=1
  Delay 1 : UnitDelay  InitialCondition=ai_layer_2_delayed_1
  mux : Mux  Inputs=1
  "pd{1,2}" : Outport
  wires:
  "p{1}"/1 -> Delay 1/1
  Delay 1/1 -> mux/1
  mux/1 -> "pd{1,2}"/1

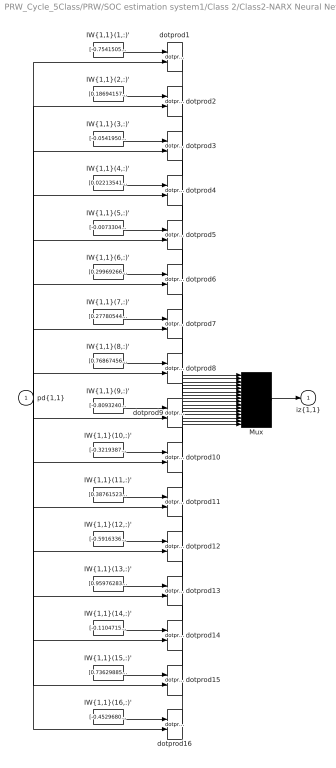
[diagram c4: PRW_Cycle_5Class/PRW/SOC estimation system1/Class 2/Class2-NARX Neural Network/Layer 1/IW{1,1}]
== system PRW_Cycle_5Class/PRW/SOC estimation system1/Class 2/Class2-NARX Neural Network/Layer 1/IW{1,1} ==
  "pd{1,1}" : Inport  PortDimensions=6  SampleTime=1
  "IW{1,1}(1,:)'" : Constant  Value=[-0.75415057701016630087309522423311136662960052490234375;-1.0602445863909493173338205451727844774723052978515625;-0.403611403758913578343481276533566415309906005859375;-0.042370088051090014358290858353939256630837917327880859375;-0.358462732167448228093320494735962711274623870849609375;0.19714157803441978433767189926584251224994659423828125]
  "IW{1,1}(10,:)'" : Constant  Value=[-0.321938743765563140097896166480495594441890716552734375;-0.368191606853078778893717526443651877343654632568359375;0.185129768716035203457437319229939021170139312744140625;0.2043650302890716308201746187478420324623584747314453125;0.8826891966589267557452558321529068052768707275390625;-0.1839543464343567913399368762839003466069698333740234375]
  "IW{1,1}(11,:)'" : Constant  Value=[0.387615236096453485981072617505560629069805145263671875;0.196254128563643603921917701882193796336650848388671875;-0.276725361207262654517080591176636517047882080078125;-0.257025784530381440351476385330897755920886993408203125;-0.64905830459941571408677418730803765356540679931640625;0.2744228849555911953217446352937258780002593994140625]
  "IW{1,1}(12,:)'" : Constant  Value=[-0.5916336524327923118704575244919396936893463134765625;0.85700047195421646950563854261417873203754425048828125;-0.2404315479020745771610023666653432883322238922119140625;-0.28768874058510063296267844634712673723697662353515625;-0.99971847270303026977700255883974023163318634033203125;1.2210817816879375730110268705175258219242095947265625]
  "IW{1,1}(13,:)'" : Constant  Value=[0.9597628331124570255639127935864962637424468994140625;-0.88562204242495046191407936930772848427295684814453125;-0.1760286219065132773398119070407119579613208770751953125;0.0927457879735908985452397246262989938259124755859375;0.722615388006634606909983631339855492115020751953125;-0.6131752174861262449923060557921417057514190673828125]
  "IW{1,1}(14,:)'" : Constant  Value=[-0.110471583141628804103362426758394576609134674072265625;0.74354882610338679516104321010061539709568023681640625;1.03451333545073875797015716671012341976165771484375;-0.3431922329775043412070090198540128767490386962890625;0.39852851406454170568594008727814070880413055419921875;1.0966067477081173908715072684572078287601470947265625]
  "IW{1,1}(15,:)'" : Constant  Value=[0.736298859452847676010378563660196959972381591796875;0.2927685967548416812178402324207127094268798828125;0.51499227548445725144432572051300667226314544677734375;-0.62644998419346598073076393120572902262210845947265625;0.923259144993893610120494486181996762752532958984375;-1.3496213250437367747736061573959887027740478515625]
  "IW{1,1}(16,:)'" : Constant  Value=[-0.452968098562966658970907474213163368403911590576171875;0.60195997671845280496683017190662212669849395751953125;1.244737450531746336679361775168217718601226806640625;-0.267275168753866976256716725401929579675197601318359375;-0.79176482905028933156899029199848882853984832763671875;-0.373843491362180591064401369294500909745693206787109375]
  "IW{1,1}(2,:)'" : Constant  Value=[0.1869415714832383390575643034026143141090869903564453125;-0.6690372979258658592272013265755958855152130126953125;0.012759415210163493892281394437304697930812835693359375;-0.1072554799884200826820546126327826641499996185302734375;0.89086845426267691205879373228526674211025238037109375;0.0110784479353181752880885824197321198880672454833984375]
  "IW{1,1}(3,:)'" : Constant  Value=[-0.054195072472333072344241600148961879312992095947265625;0.6470127629050310691383174344082362949848175048828125;0.02958524062784954888893906854718807153403759002685546875;0.0496634210674790910200471216739970259368419647216796875;-0.6458067868671537592462073007482104003429412841796875;-0.02986473920004327486932282909037894569337368011474609375]
  "IW{1,1}(4,:)'" : Constant  Value=[0.02213541632722655638776387831967440433800220489501953125;-0.240899083486367349138390636653639376163482666015625;-0.01191506308611154328624959219951051636599004268646240234375;-0.0199166550633538379233566928405707585625350475311279296875;0.239544708041063703074513568935799412429332733154296875;0.01207602017044143334623118590798185323365032672882080078125]
  "IW{1,1}(5,:)'" : Constant  Value=[-0.00733044418628346627908598520662053488194942474365234375;-0.0084764079610155744493038554310260224156081676483154296875;0.00490719146096560941694431079440619214437901973724365234375;0.004677380583939102880186577948506965185515582561492919921875;0.017297844939912286610361746852504438720643520355224609375;-0.004879080304036523436927996755230196868069469928741455078125]
  "IW{1,1}(6,:)'" : Constant  Value=[0.299692666422208875420807316913851536810398101806640625;-0.68961822746760048641334606145392172038555145263671875;0.7974891197889293348310957298963330686092376708984375;-1.4092010466297455462125753911095671355724334716796875;0.304297230825261666442571595325716771185398101806640625;0.457098009382508274622836097478284500539302825927734375]
  "IW{1,1}(7,:)'" : Constant  Value=[0.27780544103598447946978922118432819843292236328125;-1.1700995366539628239621606553555466234683990478515625;-0.63772016572320489036229673729394562542438507080078125;-0.9373334711565082244533186894841492176055908203125;-0.89278078863036325341084875617525540292263031005859375;0.5381445509060254206445961244753561913967132568359375]
  "IW{1,1}(8,:)'" : Constant  Value=[0.7686745628797455598402166287996806204319000244140625;0.90511933117887710675830703621613793075084686279296875;-0.4936655679901107429685680472175590693950653076171875;0.62958244947628572152353854107786901295185089111328125;0.8431080009011642228955452083027921617031097412109375;-0.7162116048413749158640939640463329851627349853515625]
  "IW{1,1}(9,:)'" : Constant  Value=[-0.80932403369743088905607919514295645058155059814453125;-0.91879672616566565590545678787748329341411590576171875;-0.5545659542950200915356617770157754421234130859375;-0.75253105915109508305960162033443339169025421142578125;0.5180007695523756172661933305789716541767120361328125;0.91741586556781129502269322983920574188232421875]
  Mux : Mux  Inputs=16
  dotprod{1..16} (16 alike) : neural/Weight Functions/dotprod
  "iz{1,1}" : Outport
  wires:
  "IW{1,1}(1,:)'"/1 -> dotprod1/1
  "pd{1,1}"/1 -> dotprod1/2, dotprod2/2, dotprod3/2, dotprod4/2, dotprod5/2, dotprod6/2, dotprod7/2, dotprod8/2, dotprod9/2, dotprod10/2, dotprod11/2, dotprod12/2, dotprod13/2, dotprod14/2, dotprod15/2, dotprod16/2
  dotprod1/1 -> Mux/1
  "IW{1,1}(2,:)'"/1 -> dotprod2/1
  dotprod2/1 -> Mux/2
  "IW{1,1}(3,:)'"/1 -> dotprod3/1
  dotprod3/1 -> Mux/3
  "IW{1,1}(4,:)'"/1 -> dotprod4/1
  dotprod4/1 -> Mux/4
  "IW{1,1}(5,:)'"/1 -> dotprod5/1
  dotprod5/1 -> Mux/5
  "IW{1,1}(6,:)'"/1 -> dotprod6/1
  dotprod6/1 -> Mux/6
  "IW{1,1}(7,:)'"/1 -> dotprod7/1
  dotprod7/1 -> Mux/7
  "IW{1,1}(8,:)'"/1 -> dotprod8/1
  dotprod8/1 -> Mux/8
  "IW{1,1}(9,:)'"/1 -> dotprod9/1
  dotprod9/1 -> Mux/9
  "IW{1,1}(10,:)'"/1 -> dotprod10/1
  dotprod10/1 -> Mux/10
  "IW{1,1}(11,:)'"/1 -> dotprod11/1
  dotprod11/1 -> Mux/11
  "IW{1,1}(12,:)'"/1 -> dotprod12/1
  dotprod12/1 -> Mux/12
  "IW{1,1}(13,:)'"/1 -> dotprod13/1
  dotprod13/1 -> Mux/13
  "IW{1,1}(14,:)'"/1 -> dotprod14/1
  dotprod14/1 -> Mux/14
  "IW{1,1}(15,:)'"/1 -> dotprod15/1
  dotprod15/1 -> Mux/15
  "IW{1,1}(16,:)'"/1 -> dotprod16/1
  dotprod16/1 -> Mux/16
  Mux/1 -> "iz{1,1}"/1

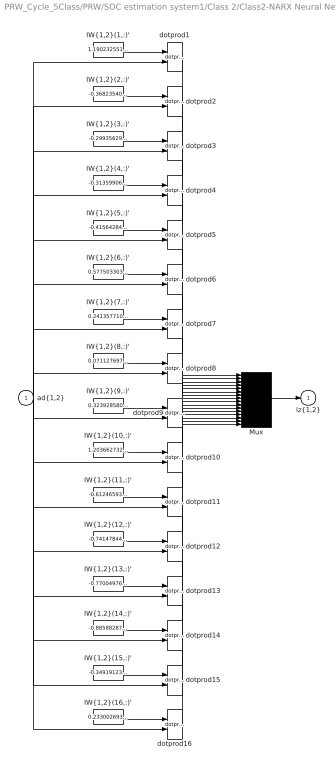
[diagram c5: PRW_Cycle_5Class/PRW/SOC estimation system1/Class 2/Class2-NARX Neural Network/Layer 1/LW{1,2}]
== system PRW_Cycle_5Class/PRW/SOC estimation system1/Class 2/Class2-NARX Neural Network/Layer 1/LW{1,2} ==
  "ad{1,2}" : Inport  PortDimensions=1  SampleTime=1
  "IW{1,2}(1,:)'" : Constant  Value=1.1902325515607079520208344547427259385585784912109375
  "IW{1,2}(10,:)'" : Constant  Value=1.2036627323236273046092037475318647921085357666015625
  "IW{1,2}(11,:)'" : Constant  Value=-0.61246593854063480222293947008438408374786376953125
  "IW{1,2}(12,:)'" : Constant  Value=-0.7414784419285955774370222570723854005336761474609375
  "IW{1,2}(13,:)'" : Constant  Value=-0.7700497660412211065050769320805557072162628173828125
  "IW{1,2}(14,:)'" : Constant  Value=-0.88588287817542854529762053061858750879764556884765625
  "IW{1,2}(15,:)'" : Constant  Value=-0.34919123068833413103817520095617510378360748291015625
  "IW{1,2}(16,:)'" : Constant  Value=0.23300269357094716138334433708223514258861541748046875
  "IW{1,2}(2,:)'" : Constant  Value=-0.368235400748596009012914009872474707663059234619140625
  "IW{1,2}(3,:)'" : Constant  Value=-0.299356293819304786207879942594445310533046722412109375
  "IW{1,2}(4,:)'" : Constant  Value=-0.313599061992354710692865182863897643983364105224609375
  "IW{1,2}(5,:)'" : Constant  Value=-0.415642846228695794774665728255058638751506805419921875
  "IW{1,2}(6,:)'" : Constant  Value=0.577503303425816572058693054714240133762359619140625
  "IW{1,2}(7,:)'" : Constant  Value=0.241357710985629025923770996087114326655864715576171875
  "IW{1,2}(8,:)'" : Constant  Value=0.07112769749609226810349582592607475817203521728515625
  "IW{1,2}(9,:)'" : Constant  Value=0.32392858033215443658292542750132270157337188720703125
  Mux : Mux  Inputs=16
  dotprod{1..16} (16 alike) : neural/Weight Functions/dotprod
  "lz{1,2}" : Outport
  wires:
  "IW{1,2}(1,:)'"/1 -> dotprod1/1
  "ad{1,2}"/1 -> dotprod1/2, dotprod2/2, dotprod3/2, dotprod4/2, dotprod5/2, dotprod6/2, dotprod7/2, dotprod8/2, dotprod9/2, dotprod10/2, dotprod11/2, dotprod12/2, dotprod13/2, dotprod14/2, dotprod15/2, dotprod16/2
  dotprod1/1 -> Mux/1
  "IW{1,2}(2,:)'"/1 -> dotprod2/1
  dotprod2/1 -> Mux/2
  "IW{1,2}(3,:)'"/1 -> dotprod3/1
  dotprod3/1 -> Mux/3
  "IW{1,2}(4,:)'"/1 -> dotprod4/1
  dotprod4/1 -> Mux/4
  "IW{1,2}(5,:)'"/1 -> dotprod5/1
  dotprod5/1 -> Mux/5
  "IW{1,2}(6,:)'"/1 -> dotprod6/1
  dotprod6/1 -> Mux/6
  "IW{1,2}(7,:)'"/1 -> dotprod7/1
  dotprod7/1 -> Mux/7
  "IW{1,2}(8,:)'"/1 -> dotprod8/1
  dotprod8/1 -> Mux/8
  "IW{1,2}(9,:)'"/1 -> dotprod9/1
  dotprod9/1 -> Mux/9
  "IW{1,2}(10,:)'"/1 -> dotprod10/1
  dotprod10/1 -> Mux/10
  "IW{1,2}(11,:)'"/1 -> dotprod11/1
  dotprod11/1 -> Mux/11
  "IW{1,2}(12,:)'"/1 -> dotprod12/1
  dotprod12/1 -> Mux/12
  "IW{1,2}(13,:)'"/1 -> dotprod13/1
  dotprod13/1 -> Mux/13
  "IW{1,2}(14,:)'"/1 -> dotprod14/1
  dotprod14/1 -> Mux/14
  "IW{1,2}(15,:)'"/1 -> dotprod15/1
  dotprod15/1 -> Mux/15
  "IW{1,2}(16,:)'"/1 -> dotprod16/1
  dotprod16/1 -> Mux/16
  Mux/1 -> "lz{1,2}"/1

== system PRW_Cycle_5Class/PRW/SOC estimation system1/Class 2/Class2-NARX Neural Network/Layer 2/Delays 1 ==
  "p{2}" : Inport  PortDimensions=16  SampleTime=1
  mux : Mux  Inputs=1
  "pd{2,1}" : Outport
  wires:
  "p{2}"/1 -> mux/1
  mux/1 -> "pd{2,1}"/1

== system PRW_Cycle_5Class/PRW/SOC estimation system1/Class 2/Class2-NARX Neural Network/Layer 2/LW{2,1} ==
  "ad{2,1}" : Inport  PortDimensions=16  SampleTime=1
  "IW{2,1}(1,:)'" : Constant  Value=[0.0007484560447357057992590068096205868641845881938934326171875;0.428302012501528384103011148908990435302257537841796875;-0.76136838015648000688173624439514242112636566162109375;-2.041090507574473189578156961943022906780242919921875;-1.5560079275295770617759671949897892773151397705078125;0.0002346400169689350358008528285580496230977587401866912841796875;0.00025834410646503381571437163444215912022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
  Mux : Mux  Inputs=1
  dotprod1 : neural/Weight Functions/dotprod
  "lz{2,1}" : Outport
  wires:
  "IW{2,1}(1,:)'"/1 -> dotprod1/1
  "ad{2,1}"/1 -> dotprod1/2
  dotprod1/1 -> Mux/1
  Mux/1 -> "lz{2,1}"/1

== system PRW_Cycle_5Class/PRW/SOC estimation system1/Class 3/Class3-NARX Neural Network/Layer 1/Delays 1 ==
  "p{1}" : Inport  PortDimensions=3  SampleTime=1
  Delay 1 : UnitDelay  InitialCondition=pi_input_1_delayed_1
  mux : Mux  Inputs=2
  "pd{1,1}" : Outport
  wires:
  "p{1}"/1 -> Delay 1/1, mux/1
  Delay 1/1 -> mux/2
  mux/1 -> "pd{1,1}"/1

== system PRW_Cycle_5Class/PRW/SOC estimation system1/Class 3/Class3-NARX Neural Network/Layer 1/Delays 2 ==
  "p{1}" : Inport  PortDimensions=1  SampleTime=1
  Delay 1 : UnitDelay  InitialCondition=ai_layer_2_delayed_1
  mux : Mux  Inputs=1
  "pd{1,2}" : Outport
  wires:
  "p{1}"/1 -> Delay 1/1
  Delay 1/1 -> mux/1
  mux/1 -> "pd{1,2}"/1
